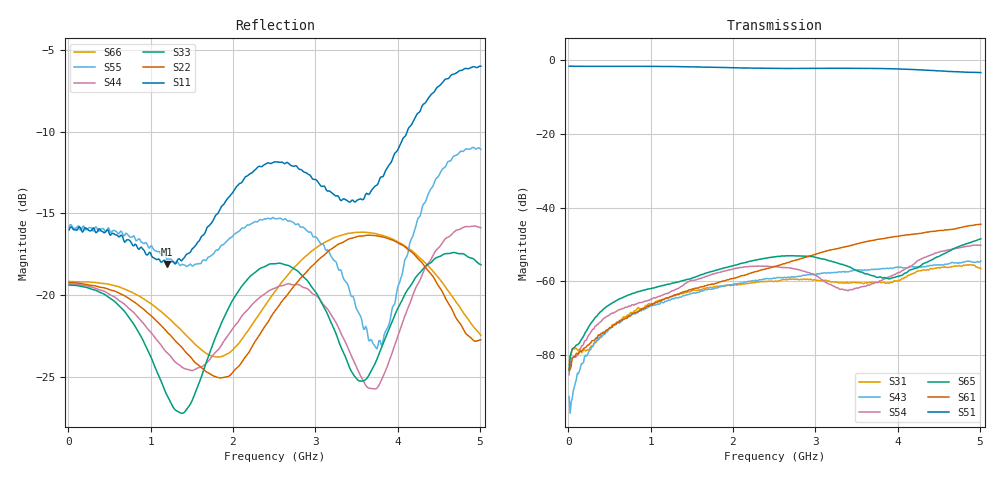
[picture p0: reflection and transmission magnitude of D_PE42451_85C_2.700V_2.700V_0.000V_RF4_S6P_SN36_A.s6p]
! Device ID: PE42451
! Serial: 36
! Insertion: A
! Temp: 85C
! VDD: 2.700
! Control_Hi: 100.000
! Control_Lo: 0.000
! Logic State: RF4
! Port 1: RFC
! Port 2: RF1
! Port 3: RF2
! Port 4: RF3
! Port 5: RF4
! Port 6: RF5
! V1 = 0.00
! V2 = 0.00
! V3 = 2.70
! V4 = 0.00
! IDD: 1.119440e-05
#  Hz  S  RI  R  50
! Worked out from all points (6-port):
!   401 points, 10 MHz to 5.01 GHz, reference 50 ohm
!   strongest paths, dB at 10 MHz, 1.26 GHz, 2.51 GHz, 3.76 GHz, 5.01 GHz:
!     S51: -1.7, -1.8, -2.3, -2.3, -3.4
!     S61: -83.6, -64.0, -55.9, -48.6, -44.5
!     S65: -84.2, -60.5, -53.3, -58.9, -48.5
!     S54: -85.3, -62.6, -56.0, -60.2, -50.3
!     S43: -91.2, -64.7, -59.2, -56.8, -54.5
!     S31: -82.4, -64.2, -60.0, -60.4, -56.5
!   lowest |S11| = -18.1 dB at 1.198 GHz (marker M1), VSWR 1.28, Z = 56.7 - j11.6 ohm
!   |S11| at or under -10 dB: start of sweep to 4.115 GHz
